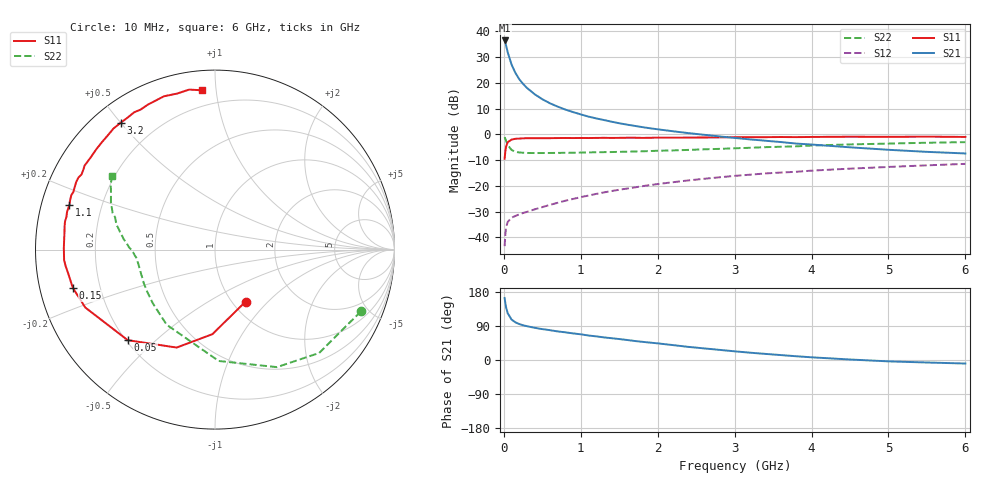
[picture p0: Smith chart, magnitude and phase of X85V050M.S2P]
! SIEMENS Small Signal Semiconductors
! BFP136W
! Si NPN RF Bipolar Junction Transistor in SOT343
! VCE = 5 V  IC = 50 mA
! Common Emitter S-Parameters:  September  1994
# GHz  S  MA  R  50
!  f  S11  S21  S12  S22
! GHz  MAG  ANG  MAG  ANG  MAG  ANG  MAG  ANG
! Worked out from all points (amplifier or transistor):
!   40 points, 10 MHz to 6 GHz, reference 50 ohm
!   highest |S21| = 36.5 dB at 10 MHz (marker M1)
!   |S21| within 3 dB of that: start of sweep to 37.55 MHz
!   unconditionally stable (mu >= 1): 715.1 MHz to 2.878 GHz
!   at 200 MHz: K = 0.53, MSG = 26.3 dB, |S12| = -31.1 dB
!   at 1.5 GHz: K = 1.11, MAG = 10.9 dB, |S12| = -21.5 dB
!   at 6 GHz: K = 0.95, MSG = 2.0 dB, |S12| = -11.5 dB
!   S11 on the Smith chart (normalised r, x): 10 MHz: 1.15, -0.75; 50 MHz: 0.21, -0.41; 150 MHz: 0.10, -0.13; 1.1 GHz: 0.08, +0.15; 3.2 GHz: 0.08, +0.50; 6 GHz: 0.11, +0.91
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0.01  0.3361 -59.4  66.94 163.7  0.0067 73.3  0.8825 -23.0
0.02  0.4717 -91.8  59.85 149.4  0.0115 62.4  0.8176 -44.8
0.03  0.5861 -111.4  52.79 138.3  0.0157 53.0  0.7402 -62.2
0.05  0.7006 -133.9  39.65 123.4  0.0198 40.9  0.6209 -88.1
0.1  0.7913 -155.9  22.81 106.9  0.024 33.3  0.4977 -122.8
0.15  0.8205 -165.0  15.68 99.4  0.0259 33.0  0.4577 -139.2
0.2  0.8268 -170.0  11.83 94.9  0.0278 34.1  0.4444 -148.5
0.25  0.8369 -173.6  9.567 91.6  0.0296 35.9  0.4391 -154.4
0.3  0.8427 -176.0  8.009 89.2  0.0311 37.8  0.4346 -158.5
0.4  0.8423 179.5  6.036 85.0  0.0348 41.2  0.4332 -163.8
0.5  0.8422 176.3  4.818 81.5  0.0385 44.6  0.4333 -167.2
0.6  0.8435 174.0  4.016 78.7  0.0426 47.3  0.4346 -169.4
0.7  0.8476 171.4  3.463 75.4  0.0467 49.7  0.4361 -170.9
0.9  0.8476 167.5  2.71 70.2  0.0555 52.5  0.4393 -173.6
1.1  0.8482 163.0  2.214 64.6  0.0646 54.6  0.445 -175.2
1.4  0.8522 157.9  1.764 57.5  0.079 55.7  0.4529 -177.3
1.6  0.8601 154.1  1.546 52.9  0.0883 55.5  0.4611 -178.8
2.2  0.8623 143.8  1.148 39.3  0.1175 53.3  0.4873 176.9
3.2  0.8806 126.7  0.798 19.3  0.1644 45.7  0.5479 168.0
4.5  0.9003 108.4  0.56 1.3  0.2155 34.3  0.6378 155.4
5.5  0.903 99.2  0.457 -6.6  0.2498 26.4  0.6873 147.7
6  0.891 94.8  0.425 -9.3  0.2669 22.1  0.706 144.3
